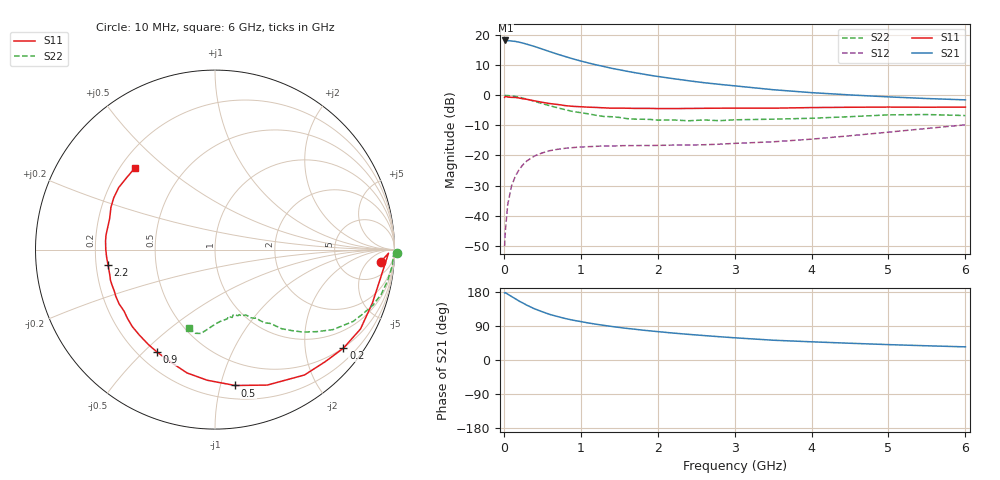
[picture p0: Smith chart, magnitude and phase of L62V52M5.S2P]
!  INFINEON TECHNOLOGIES Small Signal Semiconductors
! BFR380L3 , Si-NPN RF-Transistor in TSLP-3-1
!  Vce=2.5 V,  Ic=2.5 mA
! Common Emitter S-Parameters:  07. March 2005
#  GHz  S  MA  R  50
! f  S11  S21  S12  S22
! GHz  Mag  Ang  Mag  Ang  Mag  Ang  Mag  Ang
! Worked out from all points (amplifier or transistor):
!   36 points, 10 MHz to 6 GHz, reference 50 ohm
!   highest |S21| = 18.3 dB at 20 MHz (marker M1)
!   |S21| within 3 dB of that: start of sweep to 514.3 MHz
!   unconditionally stable (mu >= 1): 2.694 GHz to 4.666 GHz
!   at 250 MHz: K = 0.10, MSG = 20.2 dB, |S12| = -23.0 dB
!   at 1.4 GHz: K = 0.60, MSG = 12.9 dB, |S12| = -16.9 dB
!   at 6 GHz: K = 0.91, MSG = 4.1 dB, |S12| = -9.8 dB
!   S11 on the Smith chart (normalised r, x): 10 MHz: 14, -13; 200 MHz: 0.49, -2.87; 500 MHz: 0.30, -1.11; 900 MHz: 0.27, -0.55; 2.2 GHz: 0.25, -0.07; 6 GHz: 0.26, +0.40
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0.01  0.9258 -4.2  8.159 177.1  0.0031 88.1  1.015 -1.1
0.02  0.9668 -1.2  8.184 177.8  0.0056 91.3  0.9928 -2.1
0.05  0.9358 -9.7  8.138 173.8  0.0151 85.1  0.9922 -5.1
0.1  0.9261 -18.7  8.009 167.7  0.0311 79.7  0.9774 -10.1
0.15  0.9234 -28.6  7.886 161.5  0.0454 74.4  0.959 -15.0
0.2  0.9021 -37.5  7.654 155.3  0.0585 70.1  0.9337 -19.3
0.3  0.8582 -54.5  7.084 144.5  0.0813 61.7  0.8672 -27.5
0.4  0.809 -68.9  6.493 135.0  0.0983 54.6  0.7936 -34.2
0.5  0.7653 -81.6  5.878 127.3  0.1104 49.0  0.7278 -38.9
0.6  0.7292 -93.4  5.315 120.1  0.1203 44.3  0.6711 -43.2
0.7  0.7046 -102.8  4.828 114.6  0.1267 41.1  0.6207 -46.6
0.8  0.6741 -111.2  4.412 109.4  0.1318 38.3  0.5762 -49.9
0.9  0.656 -119.5  4.039 105.0  0.1352 36.2  0.5374 -51.8
1.1  0.6358 -131.5  3.456 97.6  0.1401 33.7  0.4924 -55.8
1.3  0.6198 -142.1  3.022 91.4  0.1439 32.3  0.4456 -58.8
1.6  0.6109 -154.9  2.517 83.4  0.146 31.8  0.4103 -63.9
2.2  0.602 -171.6  1.898 71.1  0.1486 35.3  0.3897 -70.7
2.8  0.6116 175.5  1.525 61.5  0.1539 41.9  0.3791 -78.8
3.5  0.6118 163.6  1.241 52.2  0.1688 49.5  0.4015 -86.0
4.5  0.6337 152.9  1.016 44.2  0.2127 60.0  0.4416 -94.7
5.5  0.6349 141.0  0.885 37.5  0.2815 64.4  0.4793 -103.4
6  0.6376 134.2  0.841 34.7  0.3235 64.0  0.4613 -108.0
